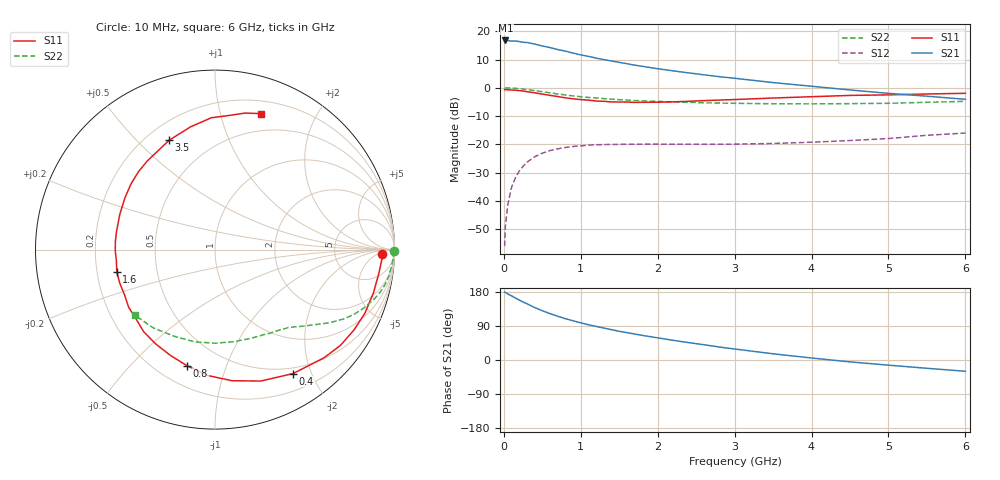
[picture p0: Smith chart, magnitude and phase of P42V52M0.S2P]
! SIEMENS Small Signal Semiconductors
! BFP182
! Si NPN RF Bipolar Junction Transistor in SOT143
! VCE = 2.5 V  IC = 2 mA
! Common Emitter S-Parameters:  March  1996
# GHz  S  MA  R  50
!  f  S11  S21  S12  S22
! GHz  MAG  ANG  MAG  ANG  MAG  ANG  MAG  ANG
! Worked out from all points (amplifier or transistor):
!   36 points, 10 MHz to 6 GHz, reference 50 ohm
!   highest |S21| = 16.7 dB at 20 MHz (marker M1)
!   |S21| within 3 dB of that: start of sweep to 670.6 MHz
!   unconditionally stable (mu >= 1): 2.179 GHz to 5.891 GHz
!   at 250 MHz: K = 0.13, MSG = 21.9 dB, |S12| = -27.7 dB
!   at 1.4 GHz: K = 0.67, MSG = 14.7 dB, |S12| = -20.0 dB
!   at 6 GHz: K = 0.98, MSG = 6.0 dB, |S12| = -16.0 dB
!   lowest NFmin = 1.10 dB at 450 MHz
!   S11 on the Smith chart (normalised r, x): 10 MHz: 24, -9; 400 MHz: 0.42, -1.73; 800 MHz: 0.32, -0.74; 1.6 GHz: 0.28, -0.10; 3.5 GHz: 0.29, +0.63; 6 GHz: 0.32, +1.35
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0.01  0.9291 -1.5  6.755 179.2  0.0016 84.5  0.9963 -0.5
0.02  0.9315 -3.2  6.866 178.4  0.0036 86.7  0.9914 -1.1
0.05  0.923 -7.9  6.851 174.5  0.0084 89.0  0.9935 -3.0
0.1  0.9154 -15.1  6.691 169.2  0.0175 79.5  0.987 -5.9
0.15  0.9075 -23.0  6.716 163.6  0.0258 76.6  0.9788 -8.9
0.2  0.8941 -30.2  6.57 158.2  0.0339 72.4  0.9672 -11.6
0.3  0.8562 -44.7  6.321 148.4  0.0485 64.5  0.9328 -16.8
0.4  0.8162 -57.8  5.929 138.5  0.0604 57.0  0.8924 -21.3
0.5  0.7754 -70.8  5.485 130.0  0.0703 50.6  0.8543 -25.0
0.6  0.7367 -82.6  5.148 122.5  0.078 45.3  0.816 -28.2
0.7  0.7029 -93.2  4.746 115.5  0.0837 40.5  0.7798 -30.8
0.8  0.6659 -103.4  4.449 109.1  0.0885 36.3  0.7481 -33.2
0.9  0.6399 -112.8  4.112 103.5  0.0923 32.9  0.7193 -35.1
1.1  0.6062 -130.9  3.59 93.0  0.0973 27.3  0.6776 -38.4
1.4  0.5634 -153.5  2.974 80.0  0.1001 20.8  0.6324 -42.8
1.6  0.561 -167.4  2.666 72.1  0.1009 18.2  0.6079 -45.4
2.2  0.5655 159.8  1.995 51.9  0.1008 13.8  0.5645 -54.0
2.8  0.6083 134.5  1.574 34.3  0.1008 12.9  0.5389 -64.1
3.5  0.6608 112.7  1.239 16.4  0.1041 14.4  0.5238 -78.3
4.5  0.7349 91.6  0.918 -5.0  0.1174 17.0  0.526 -102.4
5.5  0.7792 77.5  0.712 -21.9  0.1454 17.4  0.5555 -128.3
6  0.8002 71.2  0.627 -29.7  0.1591 14.4  0.5775 -140.9
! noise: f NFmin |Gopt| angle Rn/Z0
0.45  1.1  0.42  29  0.36
0.9  1.2  0.4  58  0.3
1.8  1.85  0.32  126  0.22
